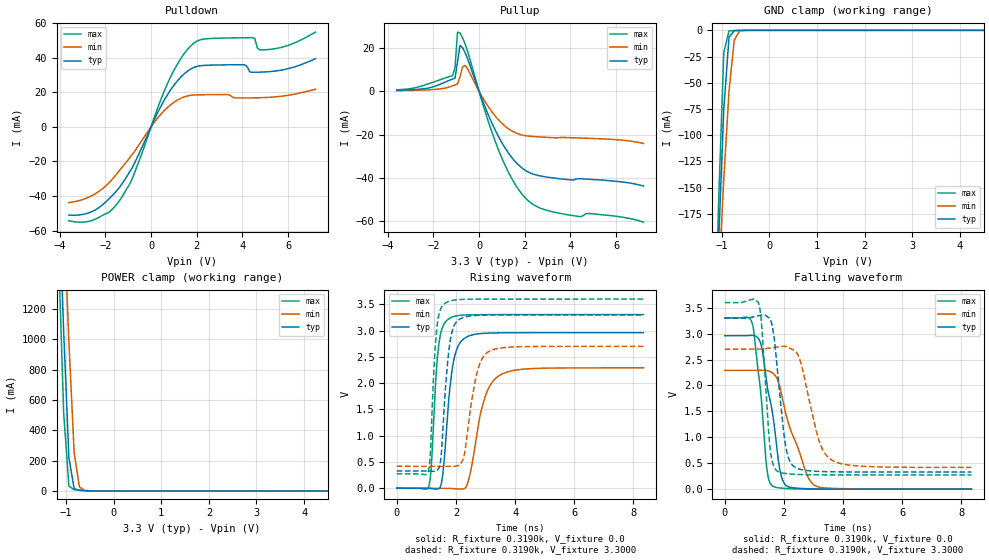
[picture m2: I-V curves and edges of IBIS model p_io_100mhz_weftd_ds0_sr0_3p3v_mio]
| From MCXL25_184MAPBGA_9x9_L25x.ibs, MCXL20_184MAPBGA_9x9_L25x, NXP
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[Model] p_io_100mhz_weftd_ds0_sr0_3p3v_mio
|   Model p_io_100mhz_weftd_ds0_sr0_3p3v_mio
| This model was characterised for following simulation conditions:
| External (pad) voltage:
|   - Typ: 3.3V,   - Min: 2.7V,   - Max: 3.6V
| Library cells for typ/min/max conditions are connected as defined below:
|  pad - External Pad
|  ipp_do_lv - Core Input
|  ipp_obe_lv - Output Buffer Enable
|  IOGC - NC
|  REFH3V3 - REFH3V3
|  REFL3V3 - REFL3V3
|  ZI - NC
|  abut_ncal_vddio[1] - vddio
|  abut_ncal_vddio[2] - vddio
|  abut_ncal_vddio[3] - vssio
|  abut_ncal_vddio[4] - vddio
|  abut_ncal_vddio[5] - vddio
|  abut_ncal_vddio[6] - vssio
|  abut_pcal_vddio[1] - vssio
|  abut_pcal_vddio[2] - vssio
|  abut_pcal_vddio[3] - vddio
|  abut_pcal_vddio[4] - vssio
|  abut_pcal_vddio[5] - vssio
|  abut_pcal_vddio[6] - vddio
|  ipp_do_1p8v - ipp_do_1p8v
|  ipp_dse_lv - 0
|  ipp_eftd_lv - NC
|  ipp_ina_mux_vddio - NC
|  ipp_ina_mux_vddio[0] - NC
|  ipp_ina_mux_vddio[1] - NC
|  ipp_ina_r0_vddio - NC
|  ipp_ina_r0a_vddio - NC
|  ipp_ina_r0b_vddio - NC
|  ipp_ina_r0c_vddio - NC
|  ipp_ina_r0d_vddio - NC
|  ipp_ina_r0e_vddio - NC
|  ipp_ina_r0f_vddio - NC
|  ipp_ina_r300_vddio - NC
|  ipp_ina_r300a_vddio - NC
|  ipp_ina_r300b_vddio - NC
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Model_type I/O
Polarity   Non-Inverting
Enable   Active-High
Vinl =   0.9900V
Vinh =   2.3100V
Vmeas =  1.6500V
Cref =   30.0000pF
Rref =   1.0000M
Vref =   3.3000V
C_comp   1.3824pF   1.3233pF   1.4661pF
|C_comp_pullup   0.6923pF   0.7238pF   0.6706pF
|C_comp_pulldown   0.6090pF   0.6618pF   0.5704pF
[Model Spec]
| variable   typ   min   max
Vinh   2.3100V   1.8900V   2.5200V
Vinl   0.9900V   0.8100V   1.0800V
[Temperature Range]   25.0000   0.1250k   -40.0000
[Voltage Range]   3.3000V   2.7000V   3.6000V
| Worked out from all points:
|   slope of the pulldown table from 0 to 0.495 V, typ, clamps not added: 36.8 ohm
|   slope of the pullup table from 0 to 0.495 V, typ, clamps not added: 37.8 ohm
|   GND clamp passes 1 mA (typ) near -0.75 V on its own axis
|   POWER clamp passes 1 mA (typ) near -0.55 V on its own axis
|   rising waveform, R_fixture 0.3190k, V_fixture 0.0: 20-80 % time 291ps typ, 502ps min, 208ps max; typ from 0 V to 2.96 V
|   rising waveform, R_fixture 0.3190k, V_fixture 3.3000: 20-80 % time 241ps typ, 386ps min, 177ps max; typ from 0.33 V to 3.3 V
|   falling waveform, R_fixture 0.3190k, V_fixture 0.0: 20-80 % time 457ps typ, 746ps min, 320ps max; typ from 2.96 V to 0 V
|   falling waveform, R_fixture 0.3190k, V_fixture 3.3000: 20-80 % time 322ps typ, 565ps min, 230ps max; typ from 3.3 V to 0.33 V
[Pulldown]
|Voltage   I(typ)   I(min)   I(max)
-3.6V     -50.99mA   -43.76mA   -54.26mA
-2.5V     -48.39mA   -39.11mA   -53.69mA
-1.4V     -35.22mA   -25.46mA   -42.92mA
-850mV    -24.19mA   -16.4mA    -30.69mA
800mV     20.23mA    12.14mA    27.32mA
1.35V     29.37mA    16.76mA    40.44mA
1.9V      34.45mA    18.38mA    48.57mA
4.1V      35.83mA    16.68mA    51.45mA
4.43V     31.54mA    16.72mA    51.52mA
4.65V     31.54mA    16.77mA    45.56mA
5.09V     31.78mA    16.98mA    44.58mA
7.2V      39.32mA    21.7mA     54.71mA
[Pullup]
|Voltage   I(typ)   I(min)   I(max)
-3.6V     392.3uA    235.2uA    607.2uA
-1.16V    5.571mA    2.41mA     7.094mA
-1.05V    6.017mA    2.857mA    10.99mA
-940mV    13.55mA    3.321mA    27.21mA
-830mV    21.12mA    6.673mA    26.77mA
-720mV    20.02mA    11.25mA    24.57mA
-610mV    17.72mA    11.8mA     21.82mA
820mV     -20.27mA   -12.85mA   -26.19mA
1.48V     -31.2mA    -18.62mA   -41.17mA
2.03V     -36.53mA   -20.52mA   -49.25mA
3.46V     -40.29mA   -21.47mA   -56.15mA
7.2V      -43.77mA   -24.12mA   -60.4mA
[GND_clamp]
|Voltage   I(typ)   I(min)   I(max)
-3.6V     -4.179A    -3.084A    -5.65A
-1.18V    -350.3mA   -344.8mA   -366.5mA
-1.07V    -203.5mA   -240.3mA   -165.6mA
-960mV    -75.17mA   -142.1mA   -21.27mA
-850mV    -6.53mA    -58.02mA   -538.4uA
-740mV    -289.9uA   -9.332mA   -209.1uA
-630mV    -85.04uA   -601.4uA   -92.54uA
-300mV    -199.1nA   -1.25uA    -48.79nA
7.2V      0A         0A         0A
[POWER_clamp]
|Voltage   I(typ)   I(min)   I(max)
-3.6V     24.55A     22.33A     26.93A
-1.16V    2.047A     2.721A     1.599A
-1.05V    1.052A     1.848A     514.6mA
-940mV    218.8mA    982.2mA    31.26mA
-830mV    15.16mA    252.6mA    8.517mA
-720mV    4.307mA    26.88mA    4.483mA
-610mV    1.728mA    3.641mA    1.672mA
7.2V      0A         0A         0A
[Ramp]
| variable   typ   min   max
dV/dt_r  1.7760/0.2909n   1.3748/0.5021n   1.9829/0.2081n
dV/dt_f  1.7821/0.3218n   1.3686/0.5645n   1.9953/0.2303n
R_load = 0.3190k
[Rising Waveform]
R_fixture= 0.3190k
V_fixture= 0.0
V_fixture_min= 0.0
V_fixture_max= 0.0
|time   V(typ)   V(min)   V(max)
0s        3.011nV    251.5nV    9.8nV
1.08ns    -136.2uV   -133.7uV   31.45mV
1.403ns   -9.863mV   462.1uV    2.652V
1.554ns   257.9mV    1.193mV    3.075V
1.748ns   1.627V     -806.3uV   3.22V
2.152ns   2.779V     -14.57mV   3.291V
2.429ns   2.896V     158.7mV    3.299V
3.011ns   2.95V      1.78V      3.304V
3.48ns    2.957V     2.149V     3.304V
8.34ns    2.96V      2.291V     3.305V
[Rising Waveform]
R_fixture= 0.3190k
V_fixture= 3.3000
V_fixture_min= 2.7000
V_fixture_max= 3.6000
|time   V(typ)   V(min)   V(max)
0s        329.6mV    418.3mV    274.4mV
1.067ns   329.7mV    418.1mV    319.9mV
1.345ns   331.6mV    418.4mV    3V
1.492ns   570mV      419.1mV    3.423V
1.639ns   1.858V     418.6mV    3.521V
1.956ns   3.114V     416.5mV    3.582V
2.259ns   3.251V     582.3mV    3.595V
2.687ns   3.29V      2.14V      3.599V
3.085ns   3.297V     2.593V     3.599V
8.34ns    3.3V       2.7V       3.6V
[Falling Waveform]
R_fixture= 0.3190k
V_fixture= 0.0
V_fixture_min= 0.0
V_fixture_max= 0.0
|time   V(typ)   V(min)   V(max)
0s        2.96V      2.291V     3.305V
935.6ps   2.967V     2.29V      3.192V
1.225ns   2.8V       2.293V     1.823V
1.421ns   2.042V     2.288V     407.2mV
1.613ns   1.48V      2.246V     61.66mV
1.84ns    454.3mV    2.021V     24.44mV
2.002ns   121.3mV    1.613V     15.48mV
2.745ns   9.966mV    329.1mV    2.309mV
3.058ns   5.239mV    67.31mV    1.158mV
8.34ns    86.65uV    196.2uV    54.92uV
[Falling Waveform]
R_fixture= 0.3190k
V_fixture= 3.3000
V_fixture_min= 2.7000
V_fixture_max= 3.6000
|time   V(typ)   V(min)   V(max)
0s        3.3V       2.7V       3.6V
1.156ns   3.349V     2.7V       3.575V
1.258ns   3.363V     2.704V     3.099V
1.531ns   3.287V     2.723V     814.5mV
1.768ns   2.378V     2.741V     352.3mV
2.062ns   828.8mV    2.753V     301.6mV
2.398ns   415mV      2.657V     285.3mV
3.181ns   342.3mV    946.9mV    276.3mV
3.592ns   335.4mV    571.7mV    275.4mV
8.34ns    329.8mV    419mV      274.5mV
